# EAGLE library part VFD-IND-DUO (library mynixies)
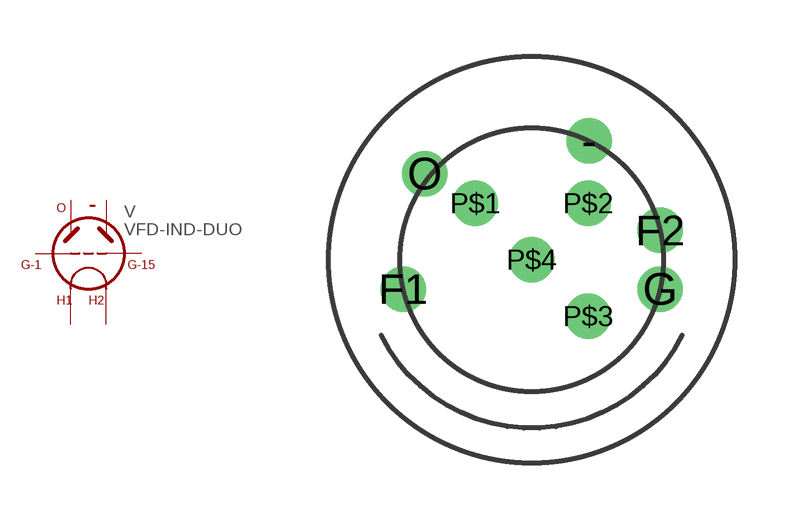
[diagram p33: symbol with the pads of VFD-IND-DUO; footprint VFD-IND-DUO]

Designator prefix V

## VFD-IND-DUO  [VFD-IND-DUO]
-  -  pas
F1  H1  pas
F2  H2  pas
G  G1  pas
O  O  pas
P$1  H1  pas
P$2  H2  pas
P$3  G15  pas
P$4  O  pas

## Footprint VFD-IND-DUO (pad centres in mm)
drill 0.7: - 1.521,3.152; F1 -3.412,-0.779; F2 3.413,0.777; G 3.412,-0.78; O -2.835,2.285; P$1 -1.5,1.5; P$2 1.5,1.5; P$3 1.5,-1.5; P$4 0,0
